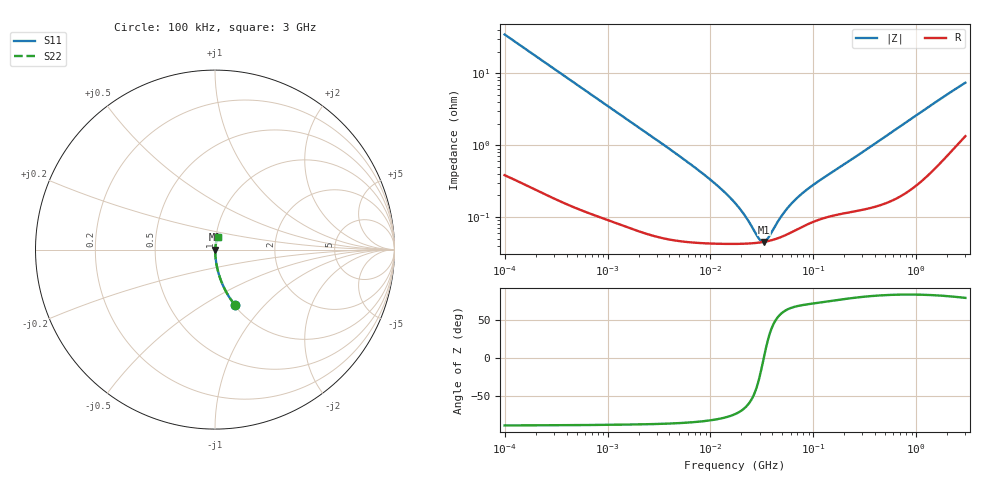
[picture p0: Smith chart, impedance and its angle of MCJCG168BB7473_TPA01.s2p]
! MCJCG168BB7473_TPA01  S-PARAMETER MODEL  ( Standard Model )
! Model Generated by TAIYO YUDEN Corporation (http://www.ty-top.com)
! Version 1.0
! TAIYO YUDEN Control No. 220601
! Copyright(c) 2015 TAIYO YUDEN CO.,LTD. All Rights Reserved.
! Product Description (link to TY-COMPAS)
! https://ds.yuden.co.jp/TYCOMPAS/or/detail?pn=MCJCG168BB7473KTPA01&u=M
! Products Name : Multilayer Ceramic Capacitors
! Characteristics :
!  Capacitance : 0.047 [uF] , Rated Voltage : 35 [V] , TCC : X7R
!  Case Size : 1.6 x 0.8 / 0.063 x 0.031 [mm/inch] , Thickness : 0.8 / 0.031 [mm/inch]
!  (Conditions: Temperature = 25 [degC] , DC Bias Voltage = 0 [V])
! External Node Assignments :
!  1  o---| |---o  2
! GND o---------o GND
! Frequency Range : 100kHz  -  3GHz  [ 401 STEP ]
# MHZ S RI R 50
! Freq[MHz].  S11 Real  S11 Imag  S21 Real  S21 Imag  S12 Real  S12 Imag  S22 Real  S22 Imag
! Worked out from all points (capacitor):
!   401 points, 100 kHz to 3 GHz, reference 50 ohm
!   read as one part in series: C = 45.6 nF near 105.3 kHz
!   lowest |Z| = 45.1 mohm at 32.99 MHz (marker M1)
!   series resonance near 32.96 MHz, so ESL is about 510 pH
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0.1  0.1109 -0.3085  0.8891 0.3085  0.8891 0.3085  0.1109 -0.3085
0.147195  0.0558 -0.2234  0.9442 0.2234  0.9442 0.2234  0.0558 -0.2234
0.228123  0.0251 -0.1494  0.9749 0.1494  0.9749 0.1494  0.0251 -0.1494
0.562235  0.00514 -0.0624  0.9949 0.0624  0.9949 0.0624  0.00514 -0.0624
1.18716  0.00172 -0.0299  0.9983 0.0299  0.9983 0.0299  0.00172 -0.0299
3.161081  0.000649 -0.0113  0.9994 0.0113  0.9994 0.0113  0.000649 -0.0113
9.574722  0.00044 -0.00345  0.9996 0.00345  0.9996 0.00345  0.00044 -0.00345
13.7349  0.000427 -0.00218  0.9996 0.00218  0.9996 0.00218  0.000427 -0.00218
17.7727  0.000425 -0.00145  0.9996 0.00145  0.9996 0.00145  0.000425 -0.00145
21.84217  0.000427 -0.000932  0.9996 0.000932  0.9996 0.000932  0.000427 -0.000932
29.75839  0.000441 -0.000226  0.9996 0.000226  0.9996 0.000226  0.000441 -0.000226
31.3325  0.000445 -0.000112  0.9996 0.000112  0.9996 0.000112  0.000445 -0.000112
32.98988  0.00045 1.81e-06  0.9995 -1.81e-06  0.9995 -1.81e-06  0.00045 1.81e-06
34.73492  0.000457 0.000116  0.9995 -0.000116  0.9995 -0.000116  0.000457 0.000116
36.57227  0.000464 0.000229  0.9995 -0.000229  0.9995 -0.000229  0.000464 0.000229
47.32384  0.00052 0.000807  0.9995 -0.000807  0.9995 -0.000807  0.00052 0.000807
58.15973  0.000592 0.00129  0.9994 -0.00129  0.9994 -0.00129  0.000592 0.00129
73.34282  0.000702 0.00185  0.9993 -0.00185  0.9993 -0.00185  0.000702 0.00185
97.38194  0.000851 0.0026  0.9991 -0.0026  0.9991 -0.0026  0.000851 0.0026
547.5153  0.00183 0.0143  0.9982 -0.0143  0.9982 -0.0143  0.00183 0.0143
1746.113  0.00771 0.0439  0.9923 -0.0439  0.9923 -0.0439  0.00771 0.0439
3000  0.0183 0.0708  0.9817 -0.0708  0.9817 -0.0708  0.0183 0.0708
